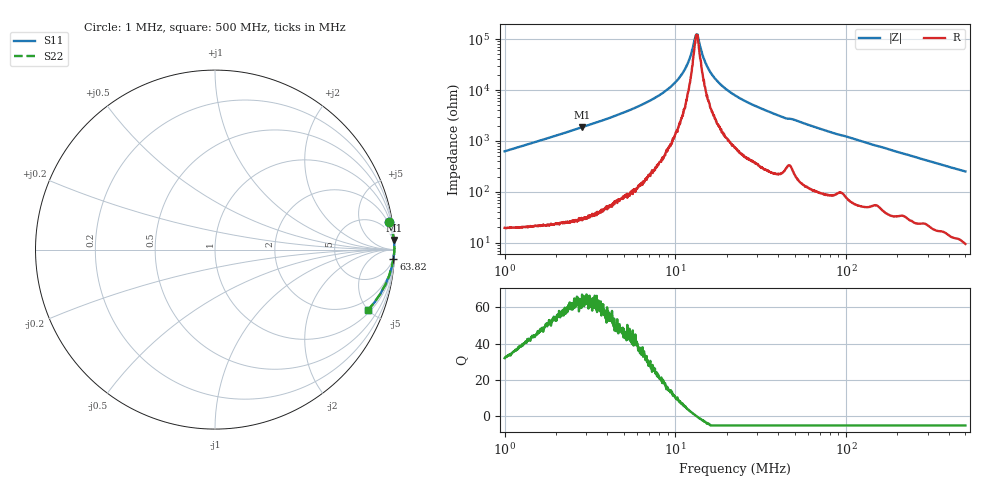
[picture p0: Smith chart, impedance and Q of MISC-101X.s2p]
!s-Parameter Generated by FASTRON Sdn. Bhd.
!FASTRON P/N : MISC-101X
!Keysight Technologies,E4991B,MY54100416,A.01.15
!Date: Thu Mar 26 11:14:26 2026
!Version  : Rev00 Thu Mar 26 11:14:26 2026
!Data & Calibration Information:
!PortZ  Port1:50+j0  Port2:50+j0
!When reading, reference impedance value at option line is always used.
! Remarks : This data is being provided solely for informational purposes.
!Freq	S11	S21	S12	S22
# Hz S dB R 50
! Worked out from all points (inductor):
!   1601 points, 1 MHz to 500 MHz, reference 50 ohm
!   read as one part in series: L = 98.9 uH near 1.032 MHz
!   highest Q = 64.5 at 2.843 MHz (marker M1), where L = 104 uH
!   self-resonance near 13.34 MHz
!   S11 on the Smith chart (normalised r, x): 1 MHz: 1, +13; 63.82 MHz: 3, -39; 500 MHz: 1.19, -5.04
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1000000  -0.15 9.0  -16.07 -79.2  -16.07 -79.2  -0.15 9.0
2820919  -0.02 3.1  -25.31 -85.9  -25.31 -85.9  -0.02 3.1
2842918  -0.02 3.1  -25.37 -86.1  -25.37 -86.1  -0.02 3.1
5354537  -0.01 1.4  -32.01 -87.3  -32.01 -87.3  -0.01 1.4
7957584  -0.01 0.7  -37.74 -86.7  -37.74 -86.7  -0.01 0.7
9663269  -0.01 0.4  -42.08 -84.6  -42.08 -84.6  -0.01 0.4
1.107042e7  -0.01 0.3  -46.82 -81.5  -46.82 -81.5  -0.01 0.3
1.201124e7  -0.01 0.1  -51.68 -73.5  -51.68 -73.5  -0.01 0.1
1.293118e7  -0.01 0.0  -59.51 -46.1  -59.51 -46.1  -0.01 0.0
1.328759e7  -0.01 0.0  -61.83 -6.1  -61.83 -6.1  -0.01 0.0
1.365382e7  -0.01 -0.0  -59.75 32.5  -59.75 32.5  -0.01 -0.0
1.436096e7  -0.01 -0.1  -54.30 64.5  -54.30 64.5  -0.01 -0.1
1.492973e7  -0.01 -0.2  -51.15 71.3  -51.15 71.3  -0.01 -0.2
1.619854e7  -0.01 -0.3  -46.61 78.4  -46.61 78.4  -0.01 -0.3
1.848541e7  -0.01 -0.4  -42.06 82.1  -42.06 82.1  -0.01 -0.4
2.236068e7  -0.01 -0.7  -37.91 83.9  -37.91 83.9  -0.01 -0.7
2.768612e7  -0.01 -1.1  -34.58 84.5  -34.58 84.5  -0.01 -1.1
3.748322e7  -0.02 -1.6  -30.83 84.5  -30.83 84.5  -0.02 -1.6
6.307767e7  -0.04 -2.9  -25.89 83.9  -25.89 83.9  -0.04 -2.9
6.381697e7  -0.04 -2.9  -25.78 83.9  -25.78 83.9  -0.04 -2.9
1.77937e8  -0.15 -8.2  -16.89 78.8  -16.89 78.8  -0.15 -8.2
5e8  -0.75 -21.3  -8.77 66.5  -8.77 66.5  -0.75 -21.3
